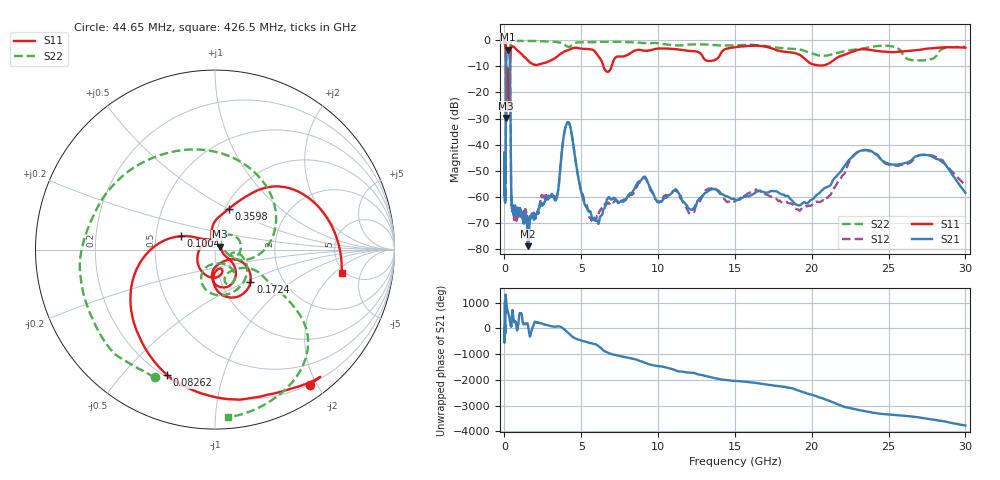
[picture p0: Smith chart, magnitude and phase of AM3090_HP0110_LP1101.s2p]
! Date/Time: Thu, Feb 28, 2019 2:00 PM
! Network Analyzer: Agilent Technologies E8364B Rev: A.07.50.67
! Sweep from 0.010 to 30.000 GHz, 1601 Points, Sweep Type: LOG
! Power Supply: 5.023 V, 0.002 A
# Hz S DB R 50
!freq MagS11 AngS11 MagS21 AngS21 MagS12 AngS12 MagS22 AngS22
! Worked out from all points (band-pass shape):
!   1601 points, 10 MHz to 30 GHz, reference 50 ohm
!   highest |S21| = -3.62 dB at 239.9 MHz (marker M1); lowest = -78.8 dB at 1.505 GHz (marker M2)
!   |S21| within 3 dB of the highest: 112.6 MHz to 344.1 MHz (231.6 MHz wide, 101 % of centre)
!   lowest |S11| = -29.8 dB at 107.7 MHz (marker M3), VSWR 1.07, Z = 52.8 + j1.78 ohm
!   |S11| at or under -10 dB: 98.38 MHz to 370.2 MHz (271.8 MHz wide, 116 % of centre); 6.447 GHz to 6.976 GHz (529 MHz wide, 7.88 % of centre)
!   |S22| runs from -27.5 to -0.1 dB; largest |S21 - S12| = 0.011
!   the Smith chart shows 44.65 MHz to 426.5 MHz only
!   S11 on the Smith chart (normalised r, x): 44.65 MHz: 0.19, -1.91; 82.62 MHz: 0.21, -0.67; 100.4 MHz: 0.68, +0.11; 172.4 MHz: 1.38, -0.53; 359.8 MHz: 1.04, +0.50; 426.5 MHz: 4.70, -2.51
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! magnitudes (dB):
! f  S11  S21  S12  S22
! 10 MHz  -0.3  -45.9  -53.2  -0.7
! 38.04 MHz  -0.5  -57.1  -59.9  -1.6
! 44.65 MHz  -0.7  -55.0  -55.8  -2.1
! 82.62 MHz  -2.5  -48.6  -50.5  -4.6
! 100.4 MHz  -13.9  -15.2  -15.3  -13.7
! 107.7 MHz  -29.8  -8.3  -8.3  -27.1
! 122.7 MHz  -13.4  -5.3  -5.2  -17.3
! 144.7 MHz  -21.9  -4.0  -4.0  -20.4
! 172.4 MHz  -11.5  -3.7  -3.7  -13.5
! 239.9 MHz  -19.2  -3.6  -3.6  -19.5
! 359.8 MHz  -12.4  -9.3  -9.2  -8.2
! 426.5 MHz  -2.9  -54.0  -52.4  -0.6
! 550.5 MHz  -2.4  -64.2  -64.3  -0.2
! 1.505 GHz  -7.6  -78.8  -68.8  -0.3
! 2.084 GHz  -9.5  -66.6  -66.5  -0.3
! 3.385 GHz  -6.4  -60.5  -60.9  -0.7
! 4.115 GHz  -3.9  -31.4  -31.4  -2.5
! 5.697 GHz  -3.6  -68.2  -69.2  -0.8
! 7.926 GHz  -5.9  -60.8  -60.6  -0.7
! 19.61 GHz  -7.5  -62.4  -63.5  -4.3
! 23.48 GHz  -3.5  -42.0  -42.1  -3.0
! 30 GHz  -2.9  -58.4  -55.3  -2.6
